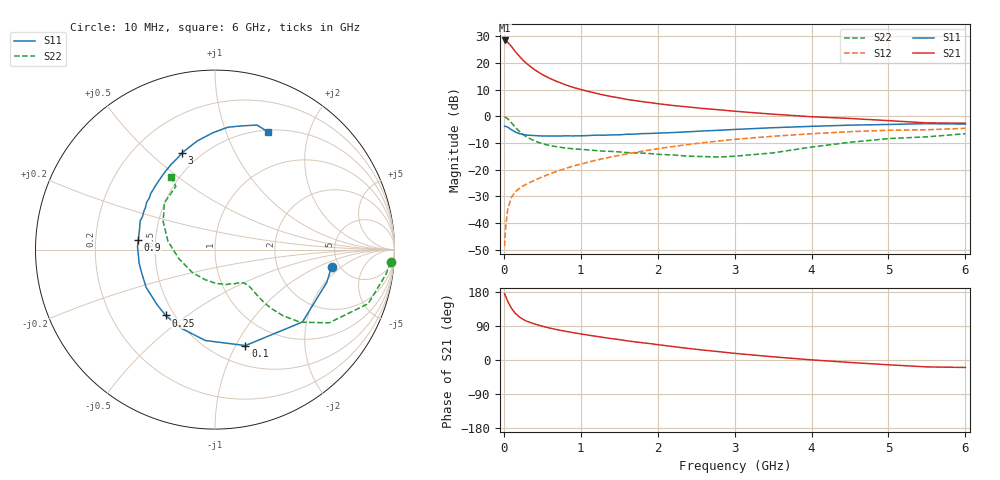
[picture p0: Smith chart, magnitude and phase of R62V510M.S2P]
! SIEMENS Small Signal Semiconductors
! BFR193
! Si NPN RF Bipolar Junction Transistor in SOT23
! VCE = 2.5 V  IC = 10 mA
! Common Emitter S-Parameters:  May  1996
# GHz  S  MA  R  50
!  f  S11  S21  S12  S22
! GHz  MAG  ANG  MAG  ANG  MAG  ANG  MAG  ANG
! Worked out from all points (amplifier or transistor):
!   36 points, 10 MHz to 6 GHz, reference 50 ohm
!   highest |S21| = 28.5 dB at 10 MHz (marker M1)
!   |S21| within 3 dB of that: start of sweep to 118.8 MHz
!   unconditionally stable (mu >= 1): 717.2 MHz to 2.014 GHz
!   at 250 MHz: K = 0.65, MSG = 23.6 dB, |S12| = -26.1 dB
!   at 1.4 GHz: K = 1.04, MAG = 10.1 dB, |S12| = -15.1 dB
!   at 6 GHz: K = 0.95, MSG = 0.9 dB, |S12| = -4.4 dB
!   lowest NFmin = 1.30 dB at 450 MHz
!   S11 on the Smith chart (normalised r, x): 10 MHz: 4.31, -1.46; 100 MHz: 0.70, -1.10; 250 MHz: 0.45, -0.42; 900 MHz: 0.40, +0.05; 3 GHz: 0.40, +0.64; 6 GHz: 0.52, +1.41
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0.01  0.657 -8.4  26.51 174.8  0.0037 85.9  0.9815 -4.1
0.02  0.6489 -16.4  26.18 169.4  0.0073 83.0  0.9626 -8.2
0.05  0.6326 -39.6  24.53 155.1  0.0182 73.5  0.9055 -19.4
0.1  0.5609 -72.4  20.37 136.2  0.0307 62.6  0.7553 -32.7
0.15  0.5094 -96.0  16.37 122.8  0.0387 57.5  0.6225 -40.5
0.2  0.4771 -113.4  13.48 113.9  0.0447 55.3  0.5274 -44.2
0.25  0.4585 -126.8  11.29 107.1  0.0498 54.9  0.4569 -46.2
0.3  0.4456 -136.2  9.687 102.2  0.0543 56.0  0.4084 -47.1
0.4  0.4376 -151.2  7.504 95.1  0.0638 57.4  0.3463 -47.3
0.5  0.4291 -161.3  6.082 89.1  0.0735 59.1  0.3085 -47.0
0.6  0.4295 -169.8  5.142 84.1  0.0841 60.8  0.2834 -47.0
0.7  0.4281 -176.6  4.453 79.7  0.0945 62.0  0.2688 -47.4
0.9  0.4306 172.9  3.507 72.3  0.1171 62.6  0.2473 -48.9
1.1  0.4375 163.4  2.934 65.6  0.1392 62.5  0.2359 -52.5
1.3  0.4441 155.5  2.513 59.4  0.163 61.9  0.2233 -56.4
1.6  0.4629 145.4  2.081 50.7  0.1986 59.9  0.2102 -64.9
2.2  0.4985 128.1  1.601 35.4  0.2727 54.0  0.1892 -87.3
3  0.57 108.7  1.251 17.5  0.3716 43.0  0.1797 -134.2
3.5  0.6142 99.1  1.1 8.4  0.4247 35.4  0.2074 -165.9
4.5  0.686 83.9  0.915 -6.5  0.5173 20.4  0.3274 151.8
5.5  0.7323 71.4  0.756 -18.2  0.5617 4.9  0.4143 121.8
6  0.7195 65.9  0.744 -19.7  0.5993 0.4  0.474 121.2
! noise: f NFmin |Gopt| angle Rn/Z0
0.45  1.3  0.22  143  0.11
0.9  1.3  0.34  160  0.11
1.8  2.05  0.54  -153  0.14
